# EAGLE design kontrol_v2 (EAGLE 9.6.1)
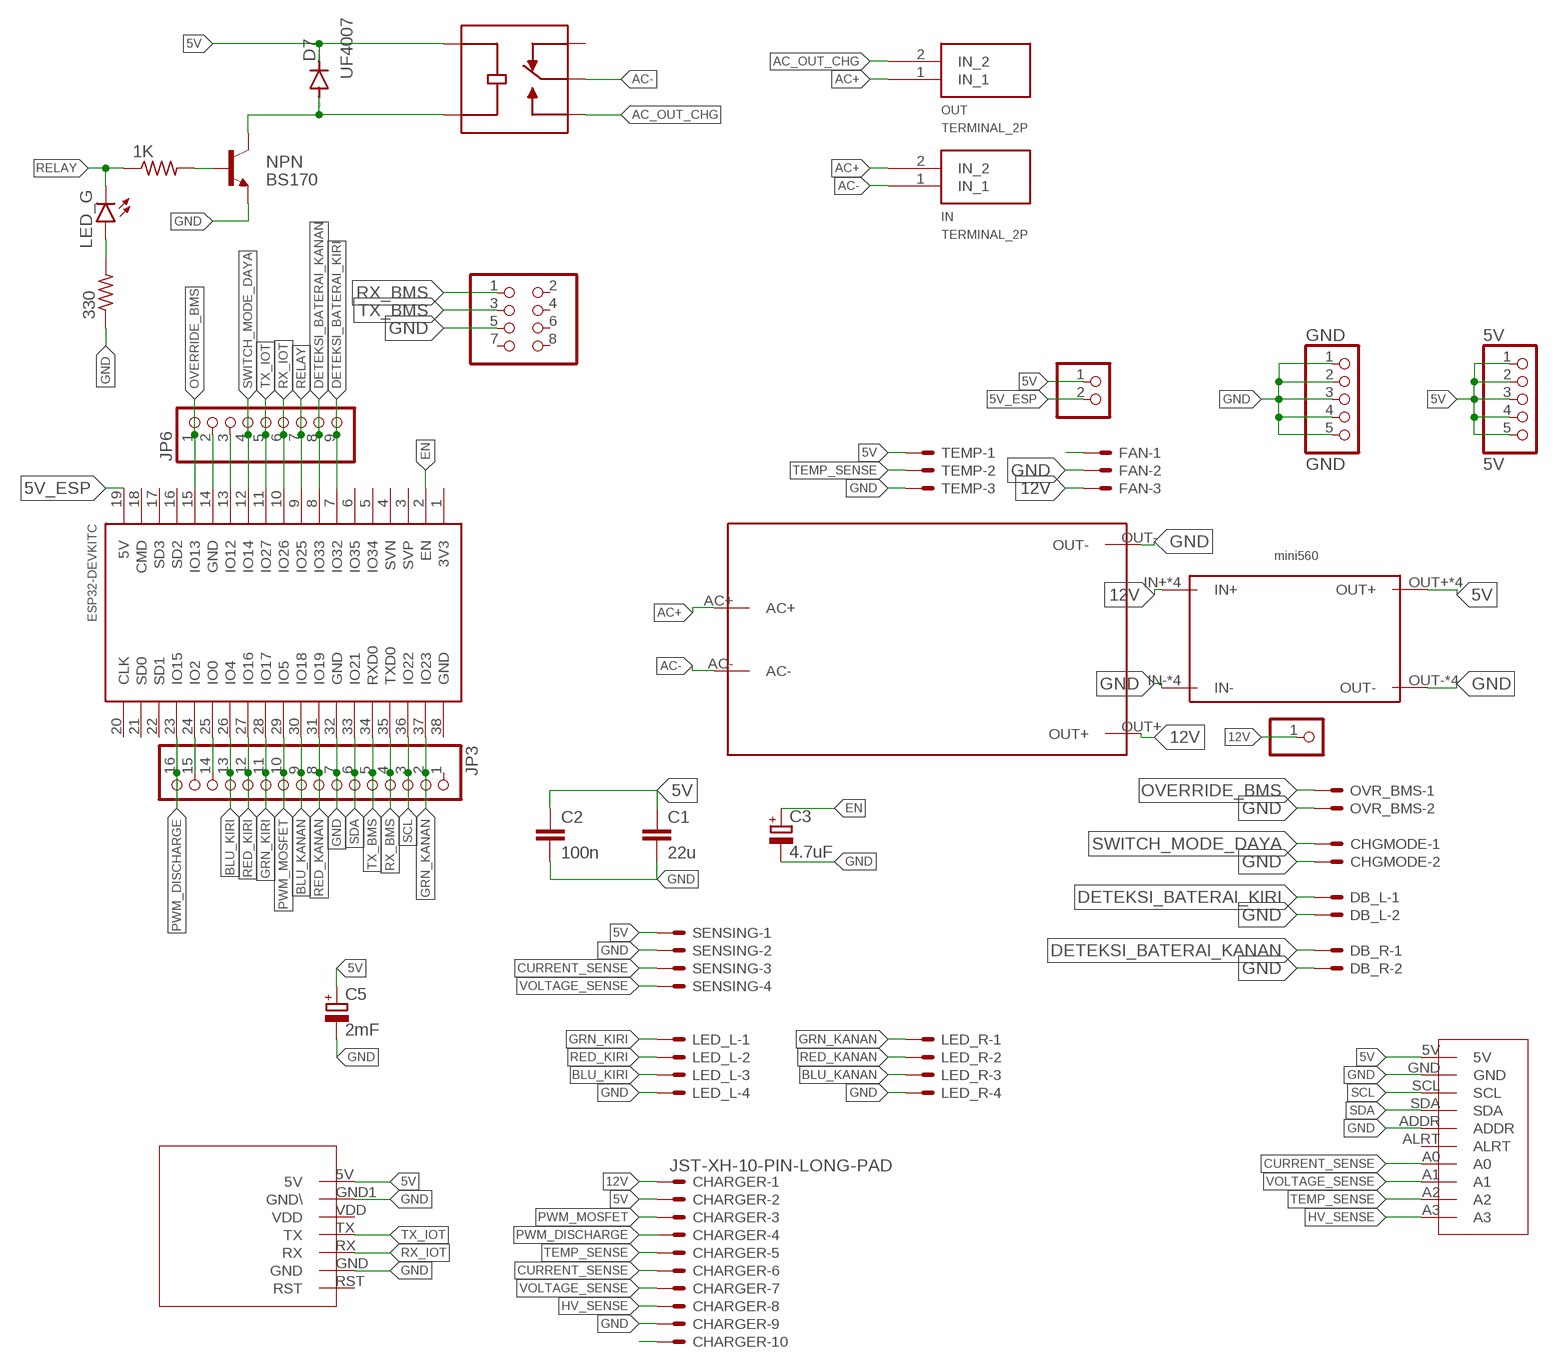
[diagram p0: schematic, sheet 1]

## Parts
1K  1k  R-US_0204/7  [0204/7]
5V  5V  PINHD-1X5  [1X05]
330  6k  R-US_0204/7  [0204/7]
C1  22u  C2.5/5  [C2.5-5]
C2  100n  C2.5/6  [C2.5-6]
C3  4.7uF  CPOL-EUE2,5-6E  [E2,5-6E]
C5  2mF  CPOL-EUE3.5-10  [E3,5-10]
CHARGER  JST-XH-10-PIN-LONG-PAD  [JST-XH-10-PACKAGE-LONG-PAD]
CHGMODE  JST-XH-02-PIN-LONG-PAD  [JST-XH-02-PACKAGE-LONG-PAD]
D4  LED_G  LED5MM  [LED_5MM]
D7  UF4007  BAS15  [DO34-7]
DB_L  JST-XH-02-PIN-LONG-PAD  [JST-XH-02-PACKAGE-LONG-PAD]
DB_R  JST-XH-02-PIN-LONG-PAD  [JST-XH-02-PACKAGE-LONG-PAD]
FAN  JST-XH-03-PIN-LONG-PAD  [JST-XH-03-PACKAGE-LONG-PAD]
GND  GND  PINHD-1X5  [1X05]
HI_LINK1  HI_LINK  [HI_LINK]
IN  TERMINAL_2P  [TERMINAL_2P]
JP2  PINHD-2X4  [2X04]
JP3  PINHD-1X16  [1X16]
JP4  PINHD-1X1  [1X01]
JP6  PINHD-1X9  [1X09]
JP7  PINHD-1X2  [1X02]
K1  SRD-12VDC-SL-C  [RELAY_SRD-12VDC-SL-C]
LED_L  JST-XH-04-PIN-LONG-PAD  [JST-XH-04-PACKAGE-LONG-PAD]
LED_R  JST-XH-04-PIN-LONG-PAD  [JST-XH-04-PACKAGE-LONG-PAD]
MINI1  MINI560  [MINI560]
NPN  BS170  BC547A-NPN-TO92-CBE  [TO92-CBE]
OUT  TERMINAL_2P  [TERMINAL_2P]
OVR_BMS  JST-XH-02-PIN-LONG-PAD  [JST-XH-02-PACKAGE-LONG-PAD]
SENSING  JST-XH-04-PIN-LONG-PAD  [JST-XH-04-PACKAGE-LONG-PAD]
TEMP  JST-XH-03-PIN-LONG-PAD  [JST-XH-03-PACKAGE-LONG-PAD]
U$1  ESP32DEVKITC  [ESP32-DEVKITC]
U$2  ADS1115  [ADS1115]
U$3  SIM800V2  [SIM800V2]

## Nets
5V: 5V.1 5V.2 5V.3 5V.4 5V.5 C1.1 C2.1 C5.+ CHARGER.2 D7.C JP7.1 K1.COIL1 MINI1.OUT+ MINI1.OUT+1(OUT+) MINI1.OUT+2(OUT+) MINI1.OUT+3(OUT+) SENSING.1 TEMP.1 U$2.5V U$3.5V
5V_ESP: JP7.2 U$1.19(5V)
12V: CHARGER.1 FAN.3 HI_LINK1.OUT+ JP4.1 MINI1.IN+ MINI1.IN+1(IN+) MINI1.IN+2(IN+) MINI1.IN+3(IN+)
AC+: HI_LINK1.AC+ IN.2(IN_2) OUT.1(IN_1)
AC-: HI_LINK1.AC- IN.1(IN_1) K1.COM
AC_OUT_CHG: K1.NO OUT.2(IN_2)
BLU_KANAN: JP3.9 LED_R.3 U$1.30(IO18)
BLU_KIRI: JP3.13 LED_L.3 U$1.26(IO4)
CURRENT_SENSE: CHARGER.6 SENSING.3 U$2.A0
DETEKSI_BATERAI_KANAN: DB_R.1 JP6.8 U$1.8(IO33)
DETEKSI_BATERAI_KIRI: DB_L.1 JP6.9 U$1.7(IO32)
EN: C3.+ U$1.2(EN)
GND: 330.1 C1.2 C2.2 C3.- C5.- CHARGER.9 CHGMODE.2 DB_L.2 DB_R.2 FAN.2 GND.1 GND.2 GND.3 GND.4 GND.5 HI_LINK1.OUT- JP2.5 JP3.7 LED_L.4 LED_R.4 MINI1.IN- MINI1.IN-1(IN-) MINI1.IN-2(IN-) MINI1.IN-3(IN-) MINI1.OUT- MINI1.OUT-1(OUT-) MINI1.OUT-2(OUT-) MINI1.OUT-3(OUT-) NPN.E OVR_BMS.2 SENSING.2 TEMP.3 U$1.32(GND) U$2.ADDR U$2.GND U$3.GND U$3.GND1(GND\)
GRN_KANAN: JP3.2 LED_R.1 U$1.37(IO23)
GRN_KIRI: JP3.11 LED_L.1 U$1.28(IO17)
HV_SENSE: CHARGER.8 U$2.A3
N$1: 330.2 D4.A
N$2: FAN.1
N$8: JP6.2 U$1.14(GND)
N$9: JP6.3 U$1.13(IO12)
N$14: CHARGER.10
N$19: 1K.2 NPN.B
N$21: D7.A K1.COIL2 NPN.C
N$23: JP3.14 U$1.25(IO0)
N$24: JP3.15 U$1.24(IO2)
OVERRIDE_BMS: JP6.1 OVR_BMS.1 U$1.15(IO13)
PWM_DISCHARGE: CHARGER.4 JP3.16 U$1.23(IO15)
PWM_MOSFET: CHARGER.3 JP3.10 U$1.29(IO5)
RED_KANAN: JP3.8 LED_R.2 U$1.31(IO19)
RED_KIRI: JP3.12 LED_L.2 U$1.27(IO16)
RELAY: 1K.1 D4.K(C) JP6.7 U$1.9(IO25)
RX_BMS: JP2.1 JP3.4 U$1.35(TXD0)
RX_IOT: JP6.6 U$1.10(IO26) U$3.RX
SCL: JP3.3 U$1.36(IO22) U$2.SCL
SDA: JP3.6 U$1.33(IO21) U$2.SDA
SWITCH_MODE_DAYA: CHGMODE.1 JP6.4 U$1.12(IO14)
TEMP_SENSE: CHARGER.5 TEMP.2 U$2.A2
TX_BMS: JP2.3 JP3.5 U$1.34(RXD0)
TX_IOT: JP6.5 U$1.11(IO27) U$3.TX
VOLTAGE_SENSE: CHARGER.7 SENSING.4 U$2.A1
Unconnected: JP2.2 JP2.4 JP2.6 JP2.7 JP2.8 JP3.1 K1.NC U$1.1(3V3) U$1.3(SVP) U$1.4(SVN) U$1.5(IO34) U$1.6(IO35) U$1.16(SD2) U$1.17(SD3) U$1.18(CMD) U$1.20(CLK) U$1.21(SD0) U$1.22(SD1) U$1.38(GND) U$2.ALRT U$3.RST U$3.VDD

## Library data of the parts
1K 330 = rcl:R-US_: RESISTOR, American symbol; SPICEPREFIX: R
5V GND = pinhead:PINHD-1X5: PIN HEADER
C1 C2 = capacitor-wima:C: CAPACITOR
C3 C5 = rcl:CPOL-EU: POLARIZED CAPACITOR, European symbol; SPICEPREFIX: C
CHARGER = Rembrandt Electronics - JST XH Connectors v1-0:JST-XH-10-PIN: JST XH Connector 2 Pin Wire to board connector. Pitch: 2,54 mm, (0.100") Number of pins: 10 Created by Rembrandt Electronics www.rembrandtelectronics.com
CHGMODE DB_L DB_R OVR_BMS = JST XH Connectors v1-0:JST-XH-02-PIN: JST XH Connector 2 Pin
D4 = Sparkfun_LED:LED: LED (Generic)
D7 = diode:BAS15: DIODE
FAN TEMP = JST XH Connectors v1-0:JST-XH-03-PIN: JST XH Connector 2 Pin Wire to board connector. Pitch: 2,54 mm, (0.100") Number of pins: 3 Created by Rembrandt Electronics www.rembrandtelectronics.com
HI_LINK1 = Hi Link:HI_LINK
IN OUT = TA_library:TERMINAL_2P
JP2 = pinhead:PINHD-2X4: PIN HEADER
JP3 = pinhead:PINHD-1X16: PIN HEADER
JP4 = pinhead:PINHD-1X1: PIN HEADER
JP6 = pinhead:PINHD-1X9: PIN HEADER
JP7 = pinhead:PINHD-1X2: PIN HEADER
K1 = TA_library:SRD-12VDC-SL-C: General Purpose Non Latching 12VDC SPDT Through Hole Relays RoHS Check availability; AVAILABILITY: Not in stock; DESCRIPTION: General Purpose Non Latching 12VDC SPDT Through Hole Relays RoHS; MF: Songle Relay; MP: SRD-12VDC-SL-C; PACKAGE: Package; PRICE: None
LED_L LED_R SENSING = JST XH Connectors v1-0:JST-XH-04-PIN: JST XH Connector 2 Pin Wire to board connector. Pitch: 2,54 mm, (0.100") Number of pins: 4 Created by Rembrandt Electronics www.rembrandtelectronics.com
MINI1 = mini560:MINI560
NPN = transistor:*-NPN-: NPN Transistror BF959 corrected 2008.03.06
U$1 = ESP32-DEVKITC:ESP32DEVKITC
U$2 = ADS1115:ADS1115
U$3 = sim800v2:SIM800V2

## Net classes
1 3A: width 3.302 mm, clearance 0.61 mm
3 HIGH Voltage: width 2.032 mm, clearance 2.54 mm
4 AC: width 2.032 mm, clearance 2.54 mm

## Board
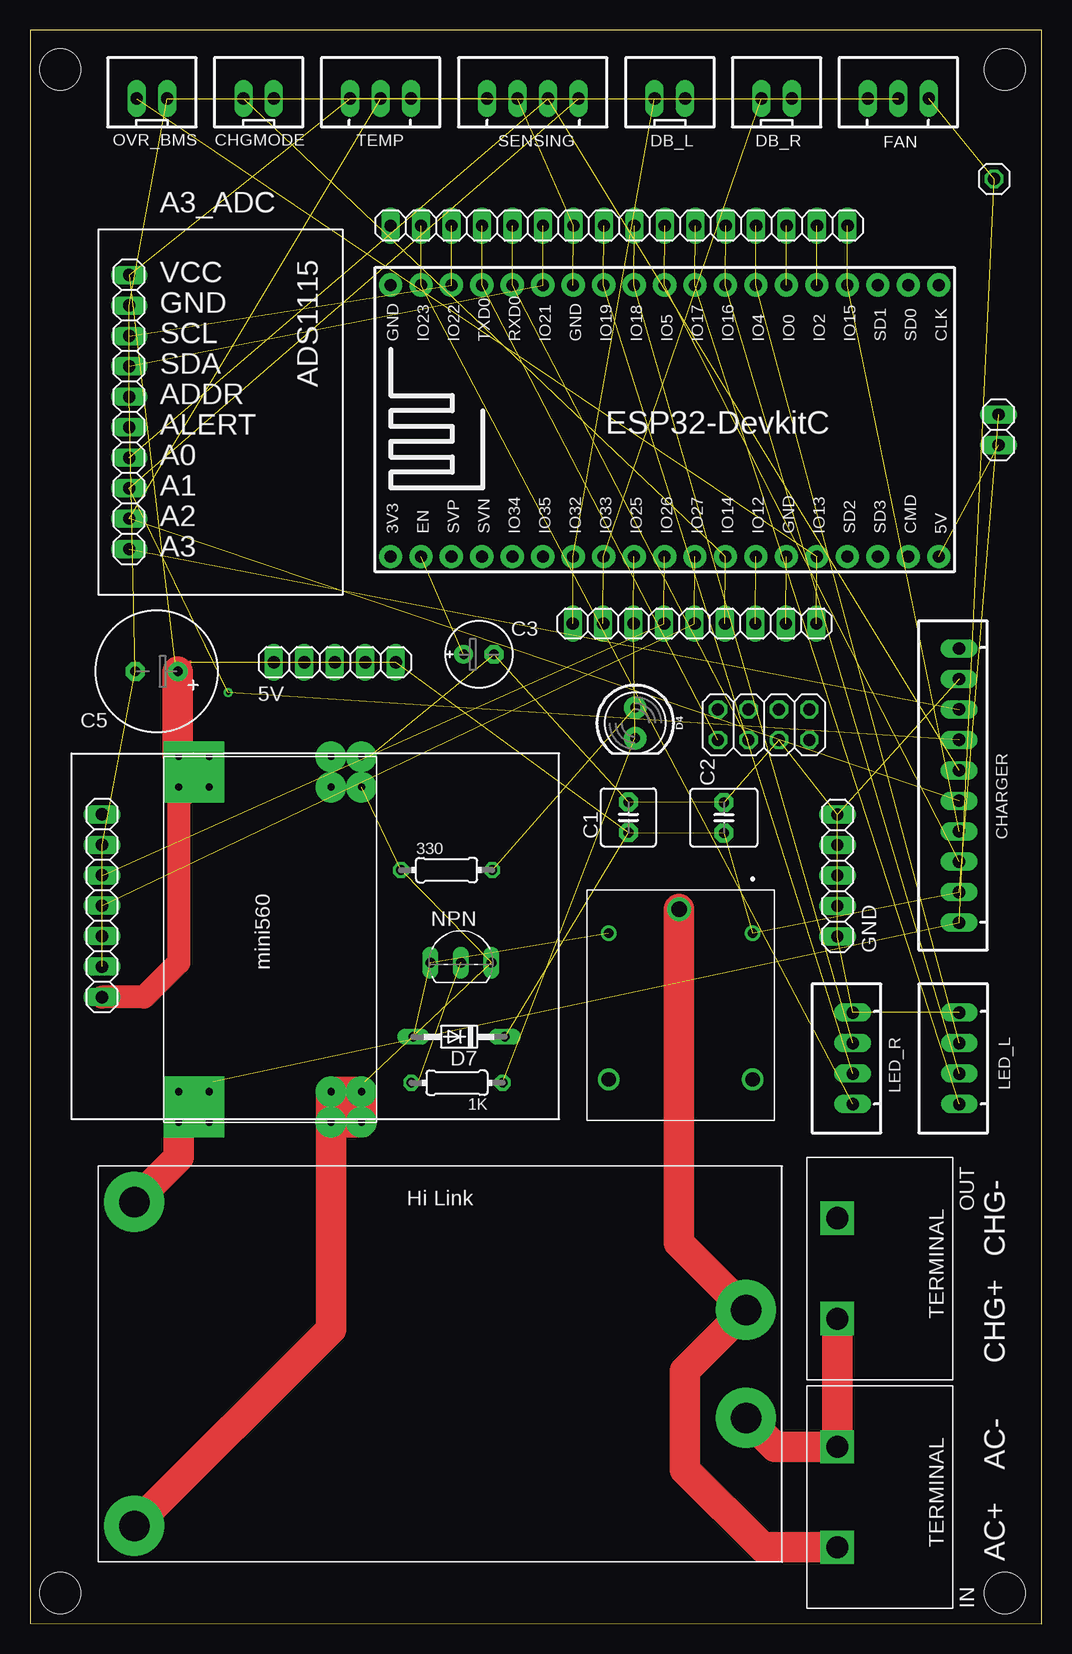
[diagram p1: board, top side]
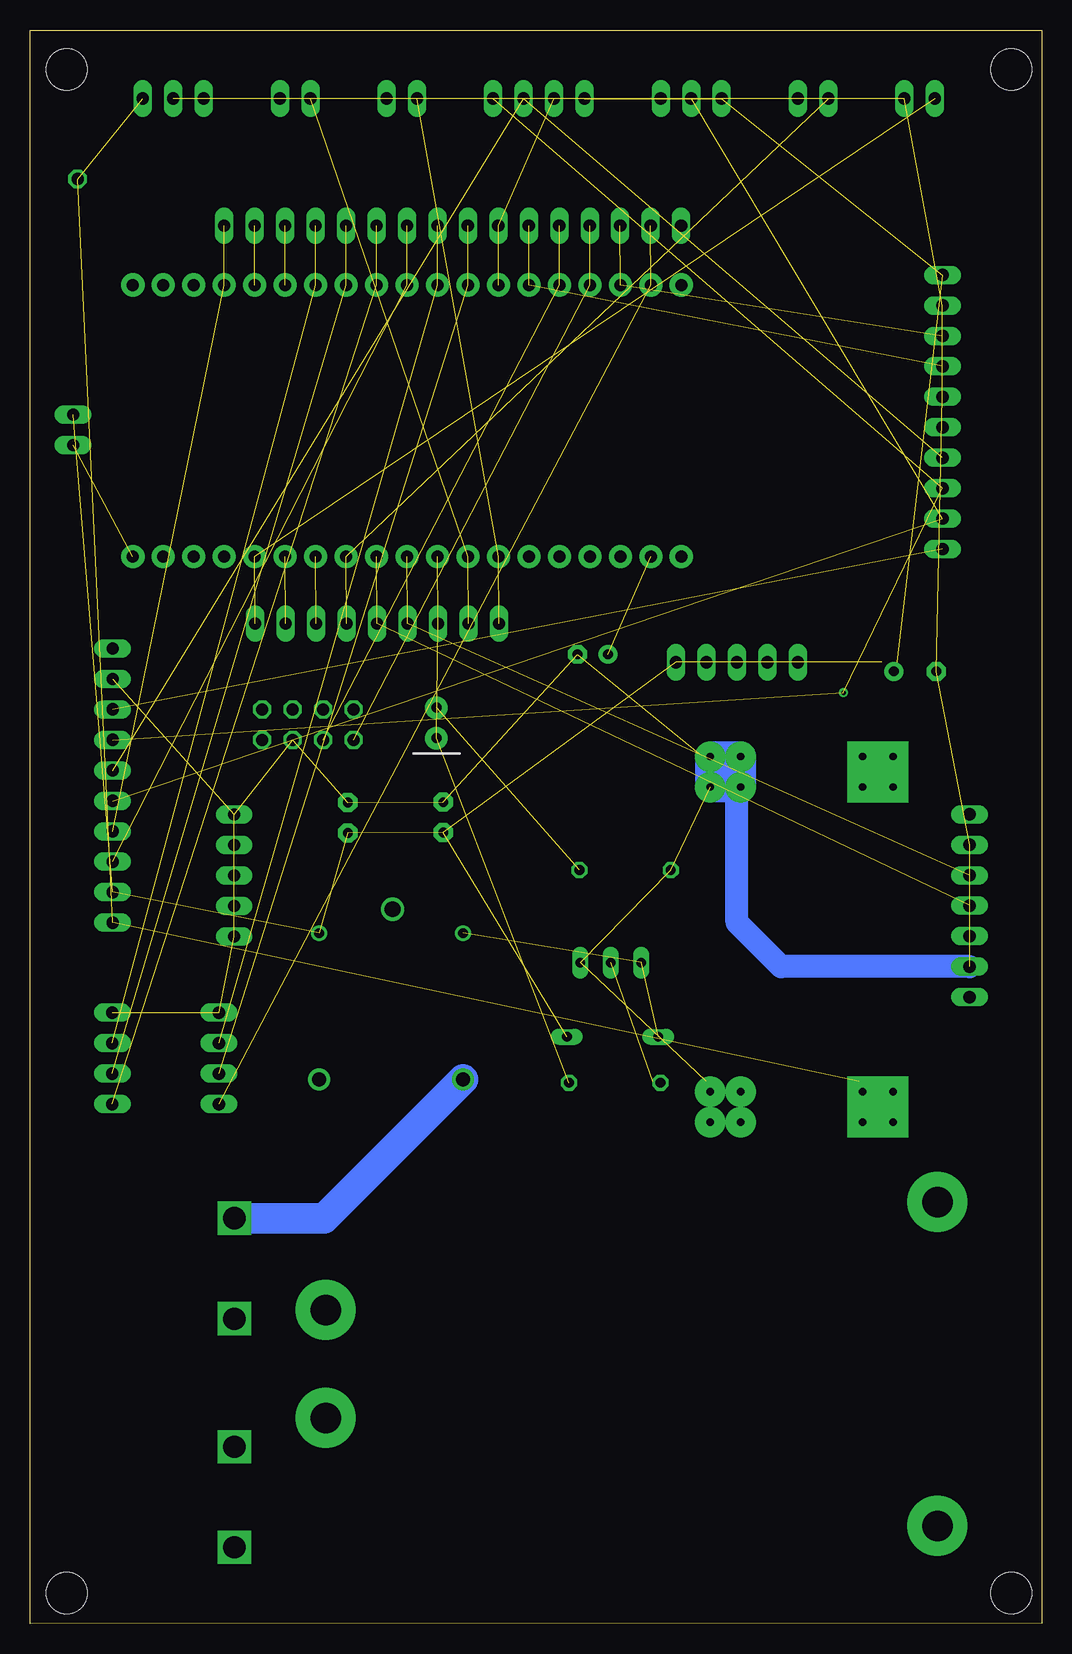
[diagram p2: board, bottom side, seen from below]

Size 84.35 x 132.84 mm. Coordinates in mm from the lower left corner, seen from the top.
Outline: 0,0.01 84.34,0 84.35,132.81 0.01,132.84 0,0.01
Copper layers (1*16): Top 0.035mm / dielectric 1.5mm / Bottom 0.035mm
Design rules "default *": minimum track width 12mil, minimum drill 0.35mm, track to track 24mil, track to pad 12mil, pad to pad 12mil, via to via 24mil, smd to smd 12mil, copper to edge 40mil, drill to drill 6mil, minimum pad ring 10mil, minimum via ring 8mil, stop-mask expansion 4mil, vias tented up to drill 0mil, thermal gap 10mil
Holes 3.4 mm at 81.27,2.55 2.53,129.55 81.27,129.55 2.53,2.55

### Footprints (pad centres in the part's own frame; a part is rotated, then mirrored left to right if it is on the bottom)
0204/7 = drill 0.813 octagon: 1 -3.81,0; 2 3.81,0
1X05 = drill 1.016 long: 1 -5.08,0; 2 -2.54,0; 3 0,0; 4 2.54,0; 5 5.08,0
C2.5-5 = drill 0.813 pad 1.6 octagon: 1 -1.27,0; 2 1.27,0
C2.5-6 = drill 0.813 pad 1.6 octagon: 1 -1.27,0; 2 1.27,0
E2,5-6E = drill 0.813 pad 1.575: + -1.27,0 | drill 0.813 pad 1.575 octagon: - 1.27,0
E3,5-10 = drill 0.813 pad 1.6: + -1.778,0 | drill 0.813 pad 1.6 octagon: - 1.778,0
JST-XH-10-PACKAGE-LONG-PAD = drill 1.016 long: 1 -11.43,0; 2 -8.89,0; 3 -6.35,0; 4 -3.81,0; 5 -1.27,0; 6 1.27,0; 7 3.81,0; 8 6.35,0; 9 8.89,0; 10 11.43,0
JST-XH-02-PACKAGE-LONG-PAD = drill 1.016 long: 1 -1.27,0; 2 1.27,0
LED_5MM = drill 0.813 pad 1.88: A -1.27,0; K 1.27,0
DO34-7 = drill 0.813 long: A 3.81,0; C -3.81,0
JST-XH-03-PACKAGE-LONG-PAD = drill 1.016 long: 1 -2.54,0; 2 0,0; 3 2.54,0
HI_LINK = drill 2.54 pad 5: AC+ -23.67,4.49; AC- -23.67,-4.51; OUT+ 27.33,-13.51; OUT- 27.33,13.49
TERMINAL_2P = drill 1.854 square: 1 0,-3.81; 2 0,4.572
2X04 = drill 1.016 octagon: 1 -3.81,-1.27; 2 -3.81,1.27; 3 -1.27,-1.27; 4 -1.27,1.27; 5 1.27,-1.27; 6 1.27,1.27; 7 3.81,-1.27; 8 3.81,1.27
1X16 = drill 1.016 long: 1 -19.05,0; 2 -16.51,0; 3 -13.97,0; 4 -11.43,0; 5 -8.89,0; 6 -6.35,0; 7 -3.81,0; 8 -1.27,0; 9 1.27,0; 10 3.81,0; 11 6.35,0; 12 8.89,0; 13 11.43,0; 14 13.97,0; 15 16.51,0; 16 19.05,0
1X01 = drill 1.016 octagon: 1 0,0
1X09 = drill 1.016 long: 1 -10.16,0; 2 -7.62,0; 3 -5.08,0; 4 -2.54,0; 5 0,0; 6 2.54,0; 7 5.08,0; 8 7.62,0; 9 10.16,0
1X02 = drill 1.016 long: 1 -1.27,0; 2 1.27,0
RELAY_SRD-12VDC-SL-C = drill 0.8: COIL1 -6.1,6; COIL2 -6.1,-6 | drill 1.3: COM -8.1,-0.12 | drill 1.2: NC 6.1,6; NO 6.1,-6
JST-XH-04-PACKAGE-LONG-PAD = drill 1.016 long: 1 -3.81,0; 2 -1.27,0; 3 1.27,0; 4 3.81,0
MINI560 = drill 0.6 pad 2.54 square: IN+ 2.54,16.51; IN+1 2.54,13.97; IN+2 0,13.97; IN+3 0,16.51; OUT+ 27.94,16.51; OUT+1 27.94,13.97; OUT+2 30.48,16.51; OUT+3 30.48,13.97 | drill 0.6 pad 2.54: IN- 2.54,1.27; IN-1 0,3.81; IN-2 2.54,3.81; IN-3 0,1.27; OUT- 27.94,1.27; OUT-1 27.94,3.81; OUT-2 30.48,3.81; OUT-3 30.48,1.27
TO92-CBE = drill 0.813 long: B 0,0; C -2.54,0; E 2.54,0
ESP32-DEVKITC = drill 1 pad 1.93: 1 -22.87,-11.42; 2 -20.33,-11.42; 3 -17.79,-11.42; 4 -15.25,-11.42; 5 -12.71,-11.42; 6 -10.17,-11.42; 7 -7.63,-11.42; 8 -5.09,-11.42; 9 -2.55,-11.42; 10 -0.01,-11.42; 11 2.53,-11.42; 12 5.07,-11.42; 13 7.61,-11.42; 14 10.15,-11.42; 15 12.69,-11.42; 16 15.23,-11.42; 17 17.77,-11.42; 18 20.31,-11.42; 19 22.85,-11.42; 20 22.85,11.23; 21 20.31,11.23; 22 17.77,11.23; 23 15.23,11.23; 24 12.69,11.23; 25 10.15,11.23; 26 7.61,11.23; 27 5.07,11.23; 28 2.53,11.23; 29 -0.01,11.23; 30 -2.55,11.23; 31 -5.09,11.23; 32 -7.63,11.23; 33 -10.17,11.23; 34 -12.71,11.23; 35 -15.25,11.23; 36 -17.79,11.23; 37 -20.33,11.23; 38 -22.87,11.23
ADS1115 = drill 1.016 long: 5V -11.43,-7.62; A0 3.81,-7.62; A1 6.35,-7.62; A2 8.89,-7.62; A3 11.43,-7.62; ADDR -1.27,-7.62; ALRT 1.27,-7.62; GND -8.89,-7.62; SCL -6.35,-7.62; SDA -3.81,-7.62
SIM800V2 = drill 1.016 long: 5V 7.62,0; GND 5.08,0; GND1 -5.08,0; RST -7.62,0; RX -2.54,0; TX 0,0; VDD 2.54,0

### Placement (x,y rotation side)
1K  35.6,45.09 180 top
5V  25.41,80.14 0 top
330  34.73,62.81 0 top
C1  49.9,67.21 90 top
C2  57.86,67.18 90 top
C3  37.43,80.8 0 top
C5  10.55,79.38 180 top
CHARGER  77.46,69.86 90 top
CHGMODE  19.06,127.13 0 top
D4  50.46,75.08 270 top
D7  35.78,48.92 180 top
DB_L  53.35,127.13 0 top
DB_R  62.24,127.13 0 top
FAN  72.4,127.13 0 top
GND  67.32,62.36 90 top
HI_LINK1  36.03,21.64 180 top
IN  67.3,10.17 0 top
JP2  61.18,74.93 0 top
JP3  49.11,116.54 0 top
JP4  80.38,120.42 0 top
JP6  55.41,83.36 180 top
JP7  80.75,99.51 270 top
K1  54.24,51.46 270 top
LED_L  77.48,47.12 90 top
LED_R  68.59,47.12 90 top
MINI1  28.91,41.79 90 top
NPN  35.93,55.09 0 top
OUT  67.3,29.22 0 top
OVR_BMS  10.17,127.13 0 top
SENSING  41.92,127.13 0 top
TEMP  29.22,127.13 0 top
U$1  52.92,100.36 0 top
U$2  15.89,100.99 270 top
U$3  6.01,59.84 270 top

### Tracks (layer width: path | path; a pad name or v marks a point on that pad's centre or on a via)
5V  (14 unrouted)
  Top 0.305: 12.08,80.14 C5.+ 13.35,80.14
  Top 1.905: MINI1.OUT+ 12.4,55.11 9.51,52.22 U$3.5V
  Top 2.54: MINI1.OUT+2 MINI1.OUT+3 MINI1.OUT+1 MINI1.OUT+ | MINI1.OUT+2 MINI1.OUT+ | MINI1.OUT+ 12.71,69.42 | C5.+ 12.33,72.34 MINI1.OUT+2
5V_ESP  (1 unrouted)
12V  (3 unrouted)
  Top 0.305: 11.44,44.58 MINI1.IN+ | 15.25,45.21 MINI1.IN+1
  Top 2.54: HI_LINK1.OUT+ 12.4,38.85 MINI1.IN+3 | MINI1.IN+3 MINI1.IN+ MINI1.IN+1 MINI1.IN+2 MINI1.IN+3
AC+
  Top 2.54: 60.72,16.13 HI_LINK1.AC+ 62.11,14.74 IN.2 OUT.1
AC-
  Top 2.54: K1.COM 54.12,31.73 HI_LINK1.AC- 54.62,21.07 54.62,12.83 61.09,6.36 IN.1
AC_OUT_CHG
  Bottom 2.54: K1.NO 59.49,34.11 59.81,33.79 OUT.2
BLU_KANAN  (2 unrouted)
BLU_KIRI  (2 unrouted)
CURRENT_SENSE  (2 unrouted)
DETEKSI_BATERAI_KANAN  (2 unrouted)
DETEKSI_BATERAI_KIRI  (2 unrouted)
EN  (1 unrouted)
GND  (28 unrouted)
  Top 0.305: 27.95,45.21 MINI1.IN-
  Top 2.54: HI_LINK1.OUT- 25.1,24.55 MINI1.IN-1 | MINI1.IN-1 MINI1.IN-2 MINI1.IN- MINI1.IN-3 MINI1.IN-1
  Bottom 0.305: 28.59,72.52 MINI1.OUT-3
  Bottom 1.905: U$3.GND 21.72,54.76 25.39,58.43 25.39,69.44 MINI1.OUT-1
  Bottom 2.54: MINI1.OUT- MINI1.OUT-1 MINI1.OUT-2 MINI1.OUT-3 MINI1.OUT-
GRN_KANAN  (2 unrouted)
GRN_KIRI  (2 unrouted)
HV_SENSE  (1 unrouted)
N$1  (1 unrouted)
N$8  (1 unrouted)
N$9  (1 unrouted)
N$19  (1 unrouted)
  Top 0.305: 32.4,45.21 1K.2
N$21  (2 unrouted)
N$23  (1 unrouted)
N$24  (1 unrouted)
OVERRIDE_BMS  (2 unrouted)
PWM_DISCHARGE  (2 unrouted)
PWM_MOSFET  (2 unrouted)
RED_KANAN  (2 unrouted)
RED_KIRI  (2 unrouted)
RELAY  (3 unrouted)
RX_BMS  (2 unrouted)
RX_IOT  (2 unrouted)
SCL  (2 unrouted)
SDA  (2 unrouted)
SWITCH_MODE_DAYA  (2 unrouted)
TEMP_SENSE  (2 unrouted)
TX_BMS  (2 unrouted)
TX_IOT  (2 unrouted)
VOLTAGE_SENSE  (via drill 0.35)  (3 unrouted)
  other vias: 16.52,77.6

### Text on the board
tNames: A3_ADC | CHG- | CHG+ | AC- | AC+

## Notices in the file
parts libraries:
Sparkfun_LED: Licensing: Creative Commons ShareAlike 4.0 International - https://creativecommons.org/licenses/by-sa/4.0
